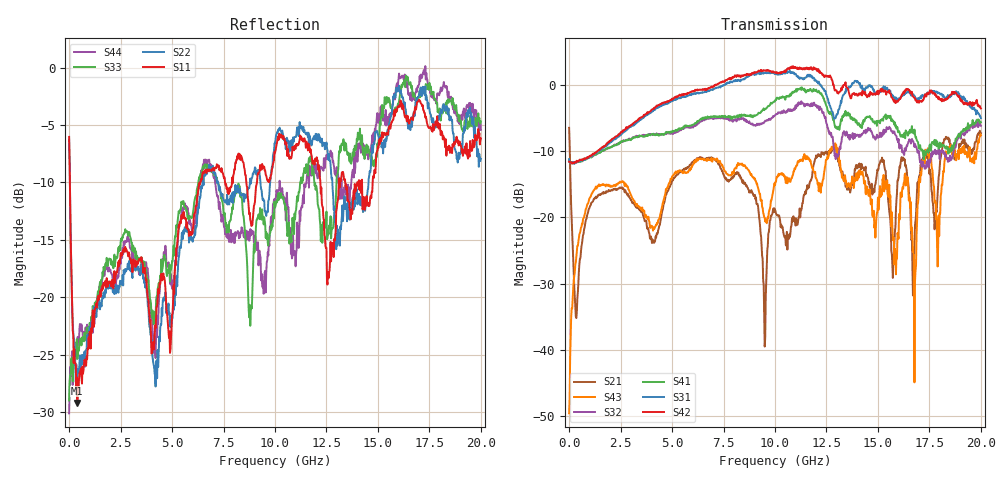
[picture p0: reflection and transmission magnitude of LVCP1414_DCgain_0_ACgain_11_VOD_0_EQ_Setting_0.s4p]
!Agilent Technologies,N5230A,MY46400459,A.07.50.48
!Agilent N5230A: A.07.50.48
!Date: Tuesday, April 17, 2012 18:36:31
!Correction: S11(Full 4 Port(1,2,3,4))
!S12(Full 4 Port(1,2,3,4))
!S13(Full 4 Port(1,2,3,4))
!S14(Full 4 Port(1,2,3,4))
!S21(Full 4 Port(1,2,3,4))
!S22(Full 4 Port(1,2,3,4))
!S23(Full 4 Port(1,2,3,4))
!S24(Full 4 Port(1,2,3,4))
!S31(Full 4 Port(1,2,3,4))
!S32(Full 4 Port(1,2,3,4))
!S33(Full 4 Port(1,2,3,4))
!S34(Full 4 Port(1,2,3,4))
!S41(Full 4 Port(1,2,3,4))
!S42(Full 4 Port(1,2,3,4))
!S43(Full 4 Port(1,2,3,4))
!S44(Full 4 Port(1,2,3,4))
!S4P File: Measurements: <S11,S12,S13,S14>,
!<S21,S22,S23,S24>,
!<S31,S32,S33,S34>,
!<S41,S42,S43,S44>:
# Hz S  dB  R 50
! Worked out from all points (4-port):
!   801 points, 300 kHz to 20 GHz, reference 50 ohm
!   strongest paths, dB at 300 kHz, 5 GHz, 10 GHz, 15 GHz, 20 GHz:
!     S42: -11.6, -2.1, 1.9, -1.1, -3.6
!     S31: -11.2, -2.5, 1.6, -1.3, -5.0
!     S41: -11.3, -7.1, -2.5, -5.4, -5.6
!     S32: -11.5, -7.3, -4.6, -8.0, -6.2
!     S43: -49.5, -13.8, -15.2, -17.0, -7.6
!     S21: -6.5, -14.5, -18.9, -12.9, -7.3
!   lowest |S11| = -29.2 dB at 400.3 MHz (marker M1), VSWR 1.07, Z = 53.2 + j1.6 ohm
!   |S11| at or under -10 dB: 37.54 MHz to 6.368 GHz (6.331 GHz wide, 198 % of centre); 12.2 GHz to 13.11 GHz (904.5 MHz wide, 7.15 % of centre); 13.41 GHz to 14 GHz (586.8 MHz wide, 4.28 % of centre)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
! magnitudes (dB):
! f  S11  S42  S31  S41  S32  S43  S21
! 300 kHz  -6.0  -11.6  -11.2  -11.3  -11.5  -49.5  -6.5
! 400.3 MHz  -29.2  -11.6  -11.6  -11.6  -11.6  -24.3  -32.2
! 7.95 GHz  -10.1  1.0  0.5  -4.8  -5.6  -13.4  -14.1
! 9.975 GHz  -7.3  1.9  1.7  -2.5  -4.7  -14.8  -18.6
! 12.73 GHz  -16.9  1.1  -3.6  -4.3  -7.3  -9.9  -9.9
! 16.78 GHz  -4.0  -2.0  -1.7  -6.8  -9.4  -44.9  -24.2
! 20 GHz  -6.2  -3.6  -5.0  -5.6  -6.2  -7.6  -7.3
